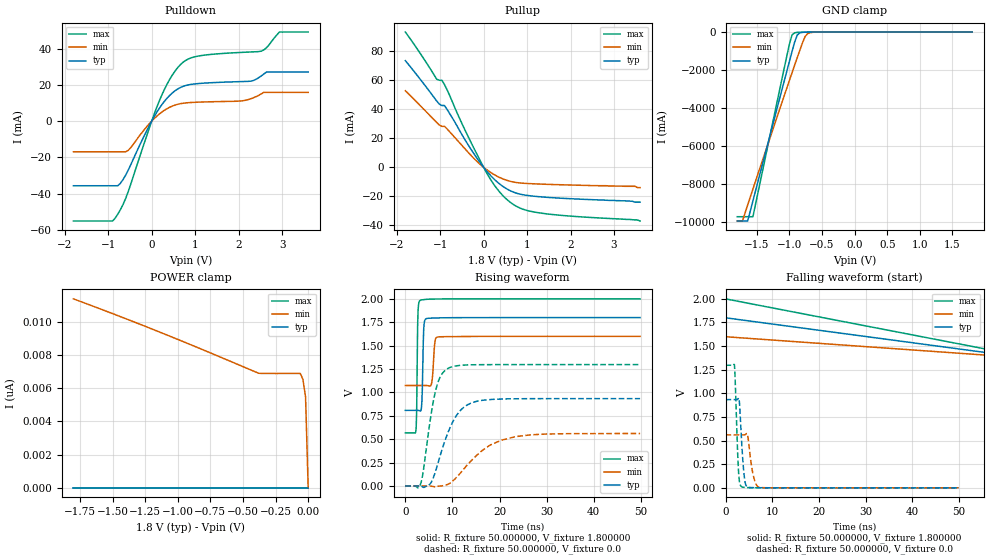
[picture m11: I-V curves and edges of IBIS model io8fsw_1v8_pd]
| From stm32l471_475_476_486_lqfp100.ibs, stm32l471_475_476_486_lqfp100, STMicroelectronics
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|   Model io8fsw_1v8_pd
[Model]  io8fsw_1v8_pd
Model_type I/O
Polarity   Non-Inverting
Enable   Active-Low
Vinl =   0.540000V
Vinh =   1.260000V
Vmeas =  0.900000V
Cref =   100.000000nF
Rref =   1.000000k
Vref =   1.800000V
C_comp   2.845500pF   2.787900pF   2.994700pF
[Temperature Range]   25.000000   0.125000k   -40.000000
[Pullup Reference]   1.800000V   1.600000V   2.000000V
[Pulldown Reference]   0.0V   0.0V   0.0V
[POWER Clamp Reference]   1.800000V   1.600000V   2.000000V
[GND Clamp Reference]   0.0V   0.0V   0.0V
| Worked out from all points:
|   slope of the pulldown table from 0 to 0.27 V, typ, clamps not added: 26.4 ohm
|   slope of the pullup table from 0 to 0.27 V, typ, clamps not added: 30.1 ohm
|   GND clamp passes 1 mA (typ) near -0.58 V on its own axis
|   rising waveform, R_fixture 50.000000, V_fixture 1.800000: 20-80 % time 264ps typ, 404ps min, 196ps max; typ from 0.808 V to 1.8 V
|   rising waveform, R_fixture 50.000000, V_fixture 0.0: 20-80 % time 4.17ns typ, 7.29ns min, 2.44ns max; typ from 0 V to 0.933 V
|   falling waveform, R_fixture 50.000000, V_fixture 1.800000: 20-80 % time 90.1ns typ, 90.1ns min, 90.1ns max; typ from 1.8 V to 0.808 V
|   falling waveform, R_fixture 50.000000, V_fixture 0.0: 20-80 % time 714ps typ, 1.02ns min, 553ps max; typ from 0.933 V to 0 V
[Pulldown]
|Voltage   I(typ)   I(min)   I(max)
-1.8V     -35.64mA   -16.93mA   -55.1mA
-840mV    -35.64mA   -16.93mA   -53.52mA
-720mV    -34.31mA   -16.93mA   -48.86mA
-540mV    -27.04mA   -16.13mA   -38.89mA
240mV     9.303mA    5.14mA     14.78mA
480mV     15.67mA    8.374mA    25.64mA
720mV     19.18mA    9.883mA    32.46mA
1.08V     20.76mA    10.49mA    35.95mA
2.1V      21.86mA    11.28mA    37.98mA
2.52V     24.95mA    15.03mA    38.63mA
2.94V     27.08mA    15.88mA    49.18mA
3.6V      27.08mA    15.88mA    49.18mA
[Pullup]
|Voltage   I(typ)   I(min)   I(max)
-1.8V     73.39mA    52.65mA    93.07mA
-1.08V    45.62mA    30.9mA     60.67mA
-960mV    42.51mA    28.16mA    59.87mA
-900mV    42.51mA    28.16mA    56.93mA
-300mV    12.8mA     8.47mA     17.72mA
60mV      -2.268mA   -1.401mA   -3.341mA
300mV     -9.801mA   -6.008mA   -14.46mA
600mV     -15.96mA   -9.582mA   -23.81mA
900mV     -18.89mA   -10.98mA   -28.81mA
1.32V     -20.37mA   -11.6mA    -31.56mA
3.48V     -24mA      -13.1mA    -36.2mA
3.6V      -24mA      -14mA      -37mA
[GND_clamp]
|Voltage   I(typ)   I(min)   I(max)
-1.8V     -9.93A     -9.932A    -9.707A
-1.72V    -9.93A     -9.932A    -9.707A
-1.64V    -9.93A     -9.083A    -9.707A
-1.56V    -8.876A    -8.251A    -9.707A
-1V       -1.54A     -2.541A    -631mA
-960mV    -1.028A    -2.139A    -153.8mA
-920mV    -527mA     -1.74A     -39.13mA
-880mV    -155.7mA   -1.344A    -18.02mA
-840mV    -45.33mA   -953mA     -12.69mA
-760mV    -8.431mA   -235mA     -7.631mA
-680mV    -3.453mA   -33.02mA   -3.876mA
1.8V      47.6uA     51.88uA    39.21uA
[POWER_clamp]
|Voltage   I(typ)   I(min)   I(max)
-1.8V     0A         11.37nA    0A
-1.14V    0A         9.374nA    0A
-380mV    0A         6.895nA    0A
-60mV     0A         6.881nA    0A
-40mV     0A         6.518nA    0A
-20mV     0A         5.452nA    0A
0V        0A         0A         0A
[Ramp]
| variable   typ   min   max
dV/dt_r  0.56008/4.16863n   0.33638/7.28484n   0.77826/2.43843n
dV/dt_f  0.59477/4.19742n   0.31494/7.40012n   0.85885/2.29079n
R_load = 50.000000
[Rising Waveform]
R_fixture= 50.000000
V_fixture= 1.800000
V_fixture_min= 1.600000
V_fixture_max= 2.000000
|time   V(typ)   V(min)   V(max)
0s        807.9mV    1.074V     568mV
2.202ns   808mV      1.074V     575.2mV
2.402ns   808mV      1.074V     801.7mV
2.703ns   807.6mV    1.074V     1.878V
3.203ns   801.3mV    1.074V     1.985V
3.504ns   891.7mV    1.074V     1.989V
3.904ns   1.68V      1.074V     1.991V
4.505ns   1.789V     1.073V     1.994V
6.807ns   1.796V     1.591V     1.998V
49.85ns   1.799V     1.599V     1.999V
[Rising Waveform]
R_fixture= 50.000000
V_fixture= 0.0
V_fixture_min= 0.0
V_fixture_max= 0.0
|time   V(typ)   V(min)   V(max)
0s        3.019nV    79.15nV    2.158nV
3.303ns   -1.625mV   -119.6nV   30.93mV
5.205ns   18.99mV    -18.46uV   677.4mV
6.406ns   156.4mV    -9.167mV   1.014V
7.508ns   342.6mV    116.5uV    1.175V
9.409ns   612.8mV    27.99mV    1.266V
11.31ns   785.3mV    117.1mV    1.287V
13.21ns   867.6mV    228.5mV    1.294V
20.42ns   928.8mV    489.5mV    1.297V
49.85ns   933.5mV    560.6mV    1.297V
[Falling Waveform]
R_fixture= 50.000000
V_fixture= 1.800000
V_fixture_min= 1.600000
V_fixture_max= 2.000000
|time   V(typ)   V(min)   V(max)
0s        1.799V     1.599V     1.999V
150.2ns   807.9mV    1.074V     568mV
300.3ns   807.9mV    1.074V     568mV
14.86us   807.9mV    1.074V     568mV
[Falling Waveform]
R_fixture= 50.000000
V_fixture= 0.0
V_fixture_min= 0.0
V_fixture_max= 0.0
|time   V(typ)   V(min)   V(max)
0s        933.5mV    560.6mV    1.297V
1.902ns   933.5mV    560.6mV    1.302V
2.803ns   950.2mV    560.6mV    157.6mV
3.003ns   884.7mV    560.6mV    57.77mV
3.504ns   438.3mV    560.4mV    10.75mV
4.004ns   124.1mV    560.4mV    5.297mV
4.404ns   23.63mV    570.3mV    4.099mV
6.106ns   1.783mV    97.96mV    1.121mV
7.207ns   1.389mV    4.469mV    768.6uV
49.85ns   3.019nV    79.15nV    2.158nV
